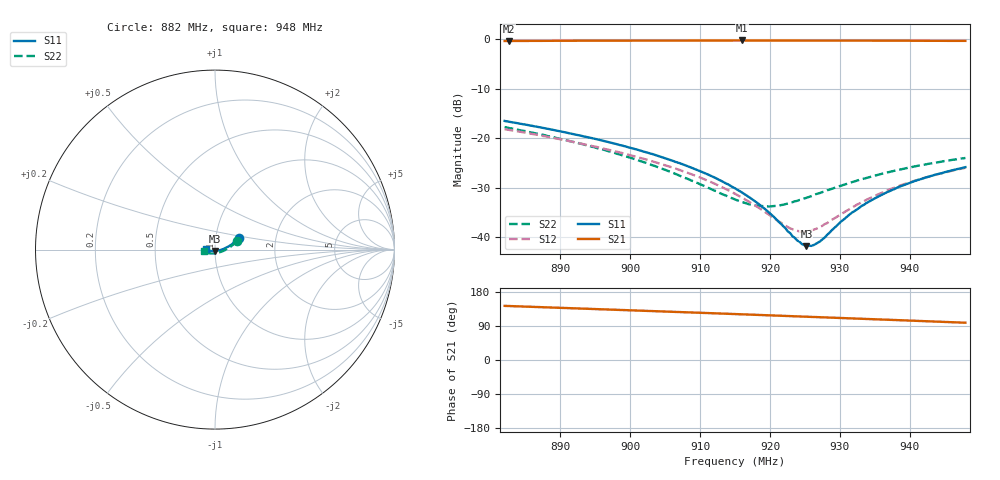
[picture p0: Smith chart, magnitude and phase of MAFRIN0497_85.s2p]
!Part Number:  MAFRIN0497
!Name:  MariaCraven
!Comments:  1
!Thu 30/Sep/2004  1:16:20 PM
!Temperature:  85
# MHZ  S  DB  R  50
!Freq  S11(dB)  S11(ang)  S21(dB)  S21(ang)  S12(dB)  S12(ang)  S22(dB)  S22(ang)
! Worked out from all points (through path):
!   201 points, 882 MHz to 948 MHz, reference 50 ohm
!   highest |S21| = -0.24 dB at 916 MHz (marker M1); lowest = -0.4 dB at 882.7 MHz (marker M2)
!   group delay of S21, straight-line fit = 1.87 ns
!   lowest |S11| = -41.8 dB at 925.2 MHz (marker M3), VSWR 1.02, Z = 50.2 - j0.8 ohm
!   |S11| at or under -10 dB: start of sweep to end of sweep
!   |S22| runs from -33.8 to -17.7 dB; largest |S21 - S12| = 0.98
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882  -16.49 26.5  -0.35 142.8  -18.15 96.2  -17.72 21.1
882.66  -16.65 26.2  -0.36 142.4  -18.31 95.7  -17.93 20.5
893.22  -19.56 19.0  -0.29 135.6  -21.15 89.8  -21.19 10.0
899.16  -21.59 14.5  -0.27 131.7  -23.08 87.5  -23.54 2.3
904.11  -23.63 10.2  -0.27 128.5  -25.06 86.4  -25.91 -6.3
910.71  -27.04 3.0  -0.25 124.1  -28.32 87.5  -29.69 -24.8
915  -30.09 -3.9  -0.24 121.3  -31.19 91.6  -32.34 -46.6
915.99  -30.92 -6.0  -0.24 120.6  -31.96 93.1  -32.85 -52.9
917.64  -32.49 -10.2  -0.26 119.4  -33.36 97.1  -33.53 -64.6
919.95  -35.09 -19.3  -0.25 117.9  -35.50 106.1  -33.77 -83.3
921.27  -36.87 -26.6  -0.26 117.0  -36.77 113.4  -33.60 -93.5
922.92  -39.16 -41.5  -0.26 115.9  -38.20 127.3  -33.00 -105.7
923.91  -40.63 -55.2  -0.26 115.2  -38.65 137.0  -32.62 -111.7
925.23  -41.77 -77.9  -0.26 114.3  -38.83 152.2  -32.02 -119.0
926.22  -41.59 -97.8  -0.26 113.6  -38.47 163.2  -31.52 -124.0
927.87  -40.01 -123.2  -0.27 112.5  -37.30 178.0  -30.69 -131.2
930.18  -36.81 -144.1  -0.27 110.9  -35.32 -167.5  -29.54 -139.1
931.83  -34.93 -152.6  -0.28 109.7  -33.93 -161.1  -28.82 -143.7
933.81  -33.07 -159.3  -0.28 108.3  -32.41 -156.2  -28.02 -148.6
937.11  -30.68 -167.0  -0.29 106.0  -30.34 -151.9  -26.79 -155.3
942.39  -27.87 -174.9  -0.31 102.3  -27.86 -149.7  -25.25 -163.4
948  -25.82 178.6  -0.33 98.4  -25.94 -150.0  -23.96 -170.7
